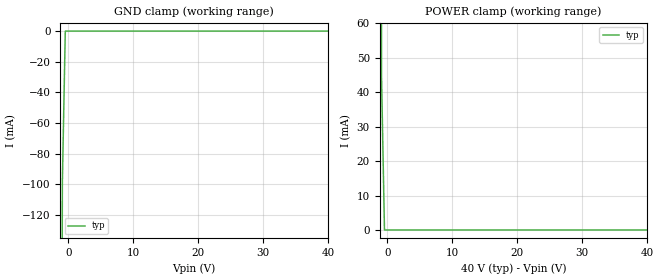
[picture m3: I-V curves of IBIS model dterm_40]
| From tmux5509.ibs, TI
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| dterm_40
[Model]   dterm_40
Model_type   Terminator
|   typ   min   max
C_comp   4.014581e-12   NA   NA
[Voltage Range]   40   NA   NA
[Temperature Range]   27   NA   NA
[Power Clamp Reference]   40   NA   NA
[GND Clamp Reference]   0   NA   NA
[GND Clamp]
-5V       -13.02A    NA         NA
-1.364V   -1.178A    NA         NA
-909.1mV  -99.73mA   NA         NA
-454.5mV  -820.3nA   NA         NA
40V       660nA      NA         NA
|   Voltage   I(typ)   I(min)   I(max)
[POWER Clamp]
|   Voltage   I(typ)   I(min)   I(max)
-5V       7.432A     NA         NA
-1.364V   581.6mA    NA         NA
-909.1mV  44.4mA     NA         NA
-454.5mV  512.7nA    NA         NA
40V       -3.008nA   NA         NA
